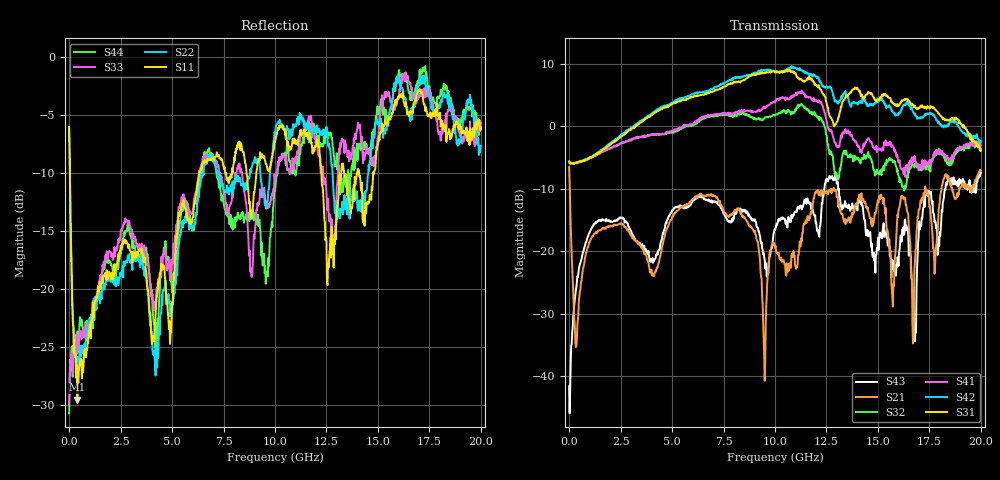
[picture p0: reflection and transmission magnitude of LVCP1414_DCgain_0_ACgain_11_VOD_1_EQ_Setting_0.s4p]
!Agilent Technologies,N5230A,MY46400459,A.07.50.48
!Agilent N5230A: A.07.50.48
!Date: Tuesday, April 17, 2012 18:29:20
!Correction: S11(Full 4 Port(1,2,3,4))
!S12(Full 4 Port(1,2,3,4))
!S13(Full 4 Port(1,2,3,4))
!S14(Full 4 Port(1,2,3,4))
!S21(Full 4 Port(1,2,3,4))
!S22(Full 4 Port(1,2,3,4))
!S23(Full 4 Port(1,2,3,4))
!S24(Full 4 Port(1,2,3,4))
!S31(Full 4 Port(1,2,3,4))
!S32(Full 4 Port(1,2,3,4))
!S33(Full 4 Port(1,2,3,4))
!S34(Full 4 Port(1,2,3,4))
!S41(Full 4 Port(1,2,3,4))
!S42(Full 4 Port(1,2,3,4))
!S43(Full 4 Port(1,2,3,4))
!S44(Full 4 Port(1,2,3,4))
!S4P File: Measurements: <S11,S12,S13,S14>,
!<S21,S22,S23,S24>,
!<S31,S32,S33,S34>,
!<S41,S42,S43,S44>:
# Hz S  dB  R 50
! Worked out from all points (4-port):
!   801 points, 300 kHz to 20 GHz, reference 50 ohm
!   strongest paths, dB at 300 kHz, 5 GHz, 10 GHz, 15 GHz, 20 GHz:
!     S31: -5.6, 3.6, 8.6, 4.2, -3.9
!     S42: -5.8, 3.8, 8.8, 4.3, -2.3
!     S41: -5.7, -0.7, 3.8, -3.6, -3.0
!     S32: -5.7, -1.0, 1.8, -7.5, -3.6
!     S21: -6.5, -14.5, -19.4, -11.8, -7.1
!     S43: -41.6, -13.4, -16.6, -17.8, -7.4
!   lowest |S11| = -29.6 dB at 400.3 MHz (marker M1), VSWR 1.07, Z = 53.1 + j1.4 ohm
!   |S11| at or under -10 dB: 37.65 MHz to 6.32 GHz (6.282 GHz wide, 198 % of centre); 12.26 GHz to 13.22 GHz (962.6 MHz wide, 7.56 % of centre); 14.08 GHz to 14.77 GHz (688.8 MHz wide, 4.77 % of centre)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
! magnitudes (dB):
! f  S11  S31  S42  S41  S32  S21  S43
! 300 kHz  -6.1  -5.6  -5.8  -5.7  -5.7  -6.5  -41.6
! 400.3 MHz  -29.6  -5.7  -5.7  -5.8  -5.8  -31.9  -24.0
! 9.95 GHz  -7.9  8.8  8.9  4.0  1.8  -19.0  -17.0
! 12.75 GHz  -14.7  1.3  5.9  -0.7  -4.4  -10.7  -8.1
! 16.78 GHz  -4.0  3.3  1.9  -4.7  -6.6  -22.8  -33.9
! 18.03 GHz  -5.2  1.7  0.4  -4.0  -4.2  -11.1  -17.5
! 20 GHz  -6.1  -3.9  -2.3  -3.0  -3.6  -7.1  -7.4
